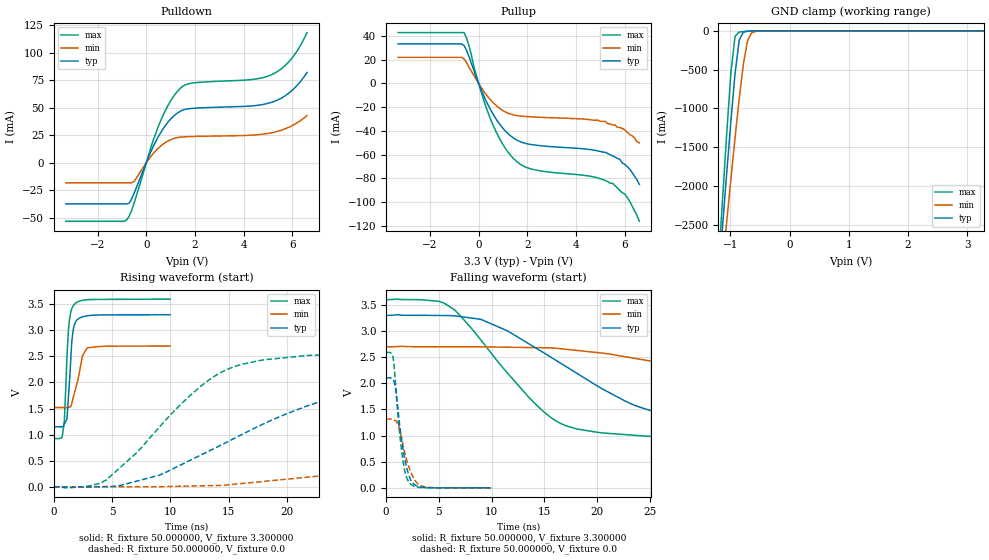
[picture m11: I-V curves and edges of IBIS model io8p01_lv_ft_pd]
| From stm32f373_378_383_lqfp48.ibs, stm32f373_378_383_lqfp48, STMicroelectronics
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|   Model io8p01_lv_ft_pd
[Model]  io8p01_lv_ft_pd
Model_type I/O
Polarity   Non-Inverting
Enable   Active-Low
Vinl =   0.990000V
Vinh =   2.310000V
Vmeas =  1.650000V
Cref =   50.000000pF
Rref =   100.000000M
Vref =   0.0V
C_comp   5.028100pF   4.857200pF   5.254400pF
[Temperature Range]   25.000000   0.125000k   -40.000000
[Pullup Reference]   3.300000V   2.700000V   3.600000V
[Pulldown Reference]   0.0V   0.0V   0.0V
[POWER Clamp Reference]   3.300000V   2.700000V   3.600000V
[GND Clamp Reference]   0.0V   0.0V   0.0V
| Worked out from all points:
|   slope of the pulldown table from 0 to 0.495 V, typ, clamps not added: 20.9 ohm
|   slope of the pullup table from 0 to 0.495 V, typ, clamps not added: 22.2 ohm
|   GND clamp passes 1 mA (typ) near -0.59 V on its own axis
|   rising waveform, R_fixture 50.000000, V_fixture 3.300000: 20-80 % time 372ps typ, 696ps min, 339ps max; typ from 1.15 V to 3.3 V
|   rising waveform, R_fixture 50.000000, V_fixture 0.0: 20-80 % time 12.6ns typ, 30.6ns min, 7.02ns max; typ from 0 V to 2.1 V
|   falling waveform, R_fixture 50.000000, V_fixture 3.300000: 20-80 % time 10.9ns typ, 23.1ns min, 6.9ns max; typ from 3.3 V to 1.15 V
|   falling waveform, R_fixture 50.000000, V_fixture 0.0: 20-80 % time 881ps typ, 1.07ns min, 738ps max; typ from 2.1 V to 0 V
[Pulldown]
|Voltage   I(typ)   I(min)   I(max)
-3.3V     -37.45mA   -18.2mA    -53.24mA
-800mV    -37.45mA   -18.2mA    -51.9mA
-700mV    -36.7mA    -18.2mA    -48.48mA
-500mV    -27.71mA   -17.01mA   -36.66mA
200mV     10.57mA    6.084mA    14.57mA
500mV     23.91mA    13.38mA    33.24mA
900mV     37.17mA    19.88mA    52.48mA
1.3V      45.55mA    23.01mA    65.5mA
1.8V      49.29mA    23.83mA    72.18mA
5.1V      54.68mA    27.07mA    79.72mA
5.9V      64.2mA     32.82mA    93.01mA
6.6V      82.13mA    42.97mA    118.5mA
[Pullup]
|Voltage   I(typ)   I(min)   I(max)
-3.3V     33.15mA    21.88mA    42.69mA
-600mV    31.87mA    20.58mA    42.69mA
-400mV    22.8mA     13.77mA    31.9mA
100mV     -5.13mA    -3.299mA   -6.952mA
500mV     -22.5mA    -14.16mA   -30.52mA
900mV     -35.28mA   -21.55mA   -48mA
1.4V      -45.54mA   -26.4mA    -62.54mA
2.2V      -51.57mA   -28.22mA   -72.25mA
4.9V      -56.8mA    -31mA      -79.6mA
5.5V      -61mA      -35mA      -84mA
6V        -68mA      -39mA      -93mA
6.6V      -85mA      -50mA      -116mA
[GND_clamp]
|Voltage   I(typ)   I(min)   I(max)
-3.3V     -9.706A    -9.438A    -9.292A
-1.2V     -3.211A    -3.571A    -3.02A
-1.13V    -2.511A    -3.008A    -2.153A
-1.06V    -1.824A    -2.453A    -1.311A
-990mV    -1.16A     -1.907A    -534mA
-920mV    -548mA     -1.377A    -70.1mA
-850mV    -120.5mA   -875.9mA   -15.92mA
-780mV    -17.67mA   -430.9mA   -9.208mA
-710mV    -5.454mA   -130.8mA   -5.036mA
-640mV    -2.091mA   -25.66mA   -2.018mA
-570mV    -553.8uA   -6.304mA   -449uA
3.28V     83.63uA    63.63uA    93.37uA
[POWER_clamp]
|Voltage   I(typ)   I(min)   I(max)
-3.28V    0A         0A         0A
0V        0A         0A         0A
[Ramp]
| variable   typ   min   max
dV/dt_r  1.26132/12.63026n   0.78882/30.58986n   1.55376/7.01157n
dV/dt_f  1.28928/10.92519n   0.70758/23.19267n   1.60433/6.88626n
R_load = 50.000000
[Rising Waveform]
R_fixture= 50.000000
V_fixture= 3.300000
V_fixture_min= 2.700000
V_fixture_max= 3.600000
|time   V(typ)   V(min)   V(max)
0s        1.15V      1.52V      925.1mV
720.7ps   1.152V     1.52V      964.7mV
900.9ps   1.204V     1.519V     1.252V
1.121ns   1.299V     1.521V     2.452V
1.341ns   2.009V     1.528V     3.199V
1.542ns   2.785V     1.605V     3.414V
1.742ns   3.087V     1.774V     3.494V
2.462ns   3.259V     2.513V     3.577V
2.863ns   3.279V     2.664V     3.587V
9.97ns    3.299V     2.699V     3.599V
[Rising Waveform]
R_fixture= 50.000000
V_fixture= 0.0
V_fixture_min= 0.0
V_fixture_max= 0.0
|time   V(typ)   V(min)   V(max)
0s        6.113nV    51.4nV     9.008nV
4.505ns   4.714mV    -214.8uV   132.3mV
9.009ns   218.5mV    1.526mV    1.134V
14.51ns   819.1mV    27.27mV    2.215V
22.02ns   1.573V     189.8mV    2.522V
28.53ns   1.909V     353.9mV    2.567V
38.54ns   2.052V     650.9mV    2.587V
58.06ns   2.096V     1.084V     2.59V
78.58ns   2.103V     1.253V     2.59V
249.2ns   2.102V     1.315V     2.59V
[Falling Waveform]
R_fixture= 50.000000
V_fixture= 3.300000
V_fixture_min= 2.700000
V_fixture_max= 3.600000
|time   V(typ)   V(min)   V(max)
0s        3.299V     2.699V     3.599V
5.005ns   3.297V     2.699V     3.567V
6.507ns   3.29V      2.699V     3.401V
11.51ns   3.002V     2.69V      2.194V
16.52ns   2.387V     2.662V     1.234V
25.03ns   1.479V     2.427V     985.8mV
32.53ns   1.277V     2.157V     949.3mV
44.54ns   1.194V     1.787V     931.7mV
68.07ns   1.155V     1.59V      925.3mV
249.2ns   1.15V      1.52V      925.1mV
[Falling Waveform]
R_fixture= 50.000000
V_fixture= 0.0
V_fixture_min= 0.0
V_fixture_max= 0.0
|time   V(typ)   V(min)   V(max)
0s        2.102V     1.315V     2.59V
660.7ps   2.068V     1.314V     2.486V
900.9ps   1.886V     1.282V     1.965V
1.161ns   1.429V     1.189V     1.293V
1.481ns   884.5mV    933mV      688.3mV
1.782ns   535.9mV    655.7mV    309.4mV
2.162ns   234.4mV    394.1mV    108.4mV
2.783ns   50.74mV    130.6mV    21.73mV
3.644ns   6.133mV    19.77mV    3.394mV
9.97ns    6.113nV    51.4nV     9.008nV
